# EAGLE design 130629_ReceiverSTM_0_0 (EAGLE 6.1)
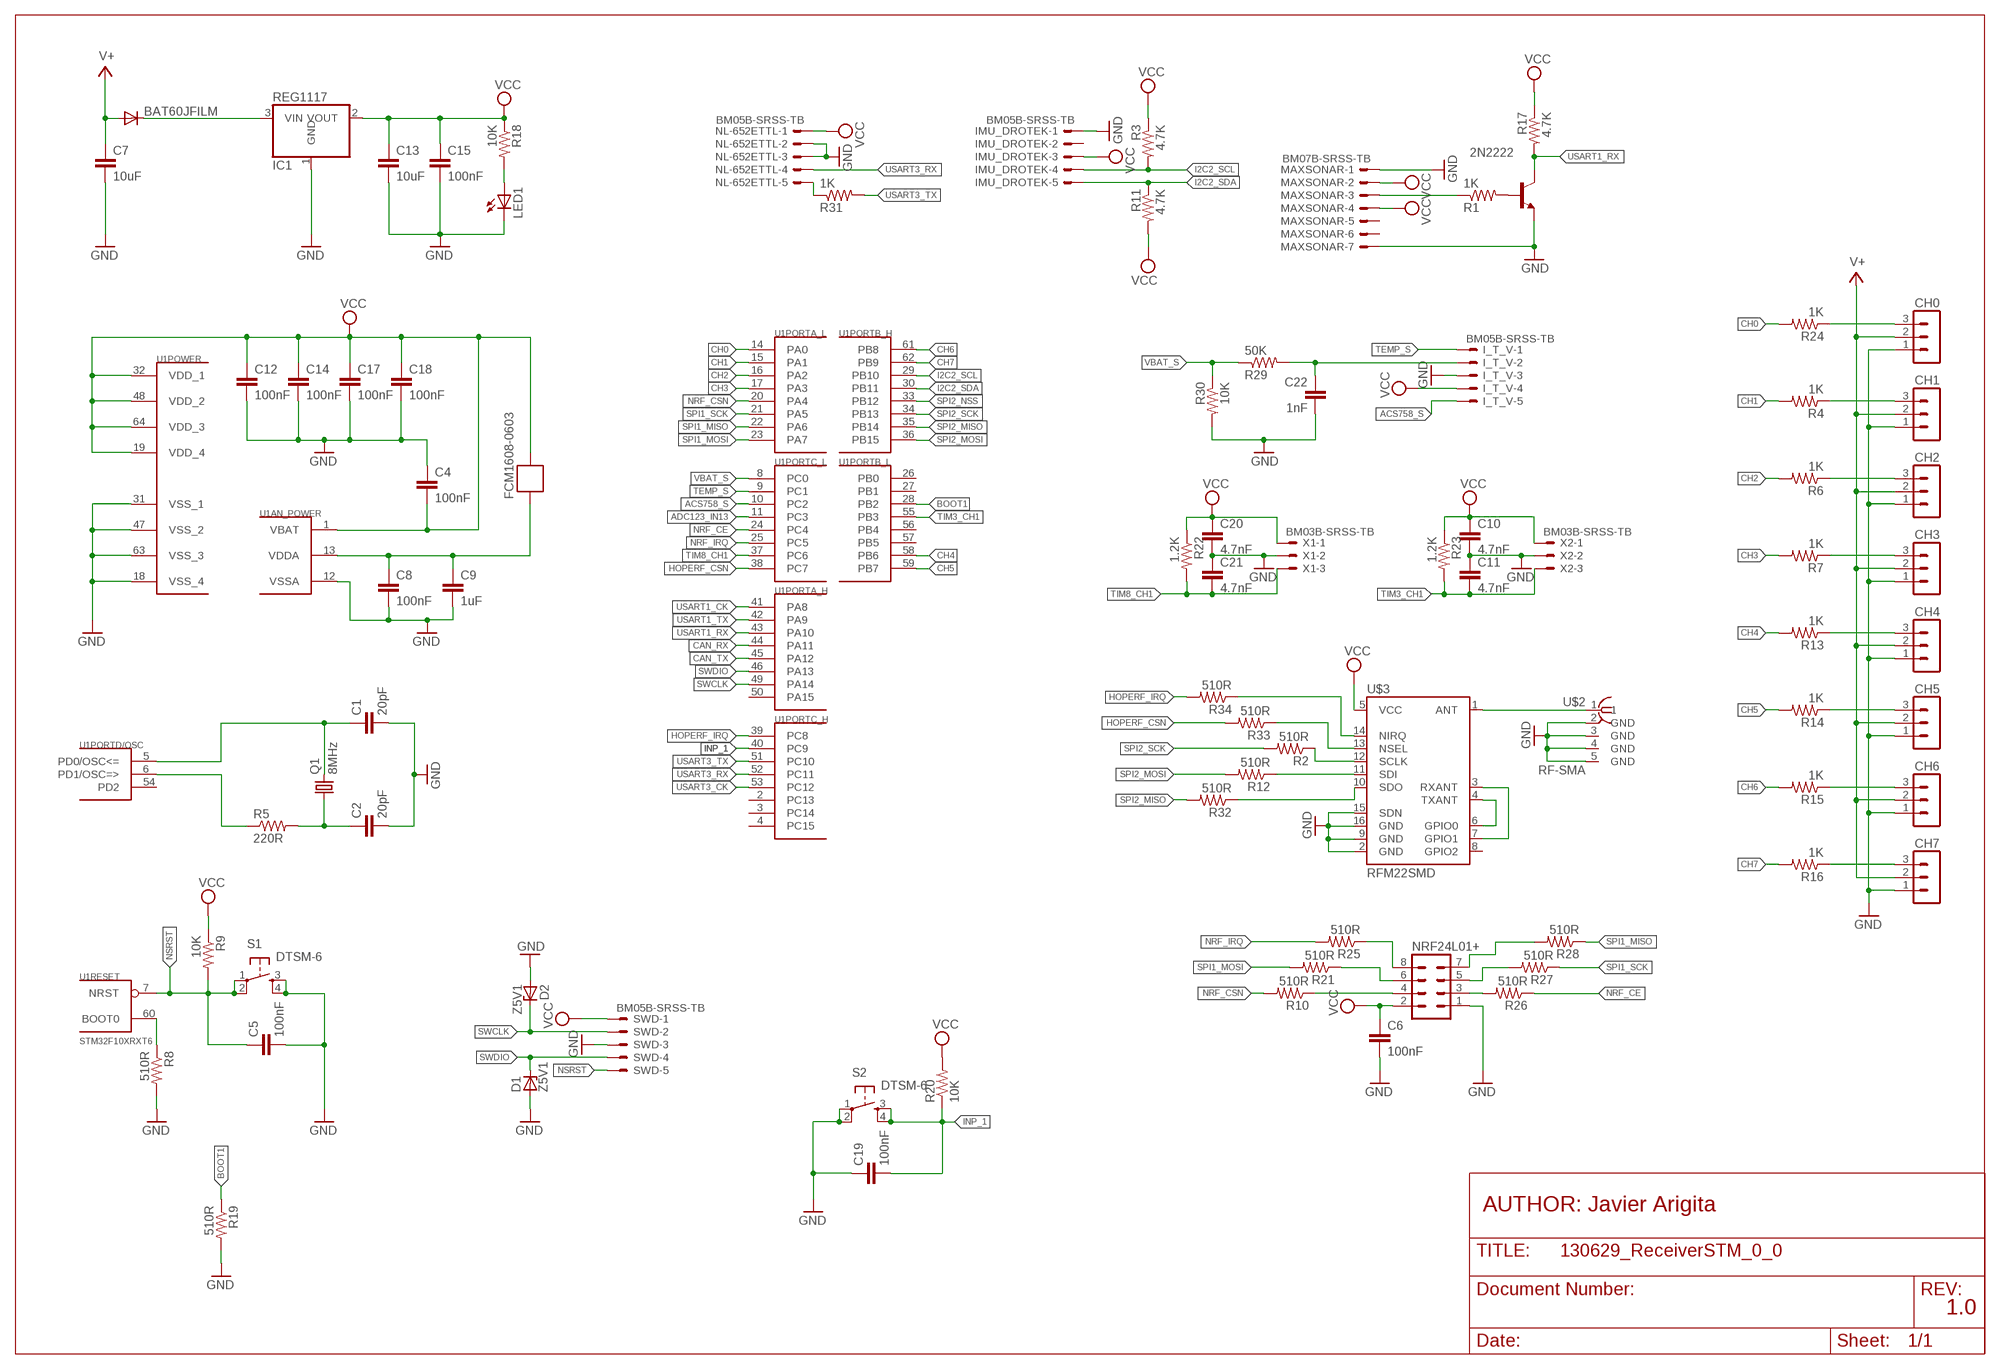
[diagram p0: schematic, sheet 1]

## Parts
2N2222  MMBT2222ALT1-NPN-SOT23-BEC  [SOT23-BEC]
BAT60JFILM  DIODE-SOD323-R  [SOD323-R]
C1  20pF  C-EUC0805  [C0805]
C2  20pF  C-EUC0805  [C0805]
C4  100nF  C-EUC0805  [C0805]
C5  100nF  C-EUC0805  [C0805]
C6  100nF  C-EUC0805  [C0805]
C7  10uF  C-EUC3216  [C3216]
C8  100nF  C-EUC0805  [C0805]
C9  1uF  C-EUC3216  [C3216]
C10  4.7nF  C-EUC0805  [C0805]
C11  4.7nF  C-EUC0805  [C0805]
C12  100nF  C-EUC0805  [C0805]
C13  10uF  C-EUC3216  [C3216]
C14  100nF  C-EUC0805  [C0805]
C15  100nF  C-EUC0805  [C0805]
C17  100nF  C-EUC0805  [C0805]
C18  100nF  C-EUC0805  [C0805]
C19  100nF  C-EUC0805  [C0805]
C20  4.7nF  C-EUC0805  [C0805]
C21  4.7nF  C-EUC0805  [C0805]
C22  1nF  C-EUC0805  [C0805]
CH0  MA03-1  [MA03-1]
CH1  MA03-1  [MA03-1]
CH2  MA03-1  [MA03-1]
CH3  MA03-1  [MA03-1]
CH4  MA03-1  [MA03-1]
CH5  MA03-1  [MA03-1]
CH6  MA03-1  [MA03-1]
CH7  MA03-1  [MA03-1]
D1  Z5V1  ZENER-DIODESOD80C  [SOD80C]
D2  Z5V1  ZENER-DIODESOD80C  [SOD80C]
FCM1608-0603  FERRITE-BEAD  [R0603]
I_T_V  BM05B-SRSS-TB  [BM05B-SRSS-TB]
IC1  REG1117  [SOT223]
IMU_DROTEK  BM05B-SRSS-TB  [BM05B-SRSS-TB]
LED1  LED0805  [CHIPLED_0805]
MAXSONAR  BM07B-SRSS-TB  [BM07B-SRSS-TB]
NL-652ETTL  BM05B-SRSS-TB  [BM05B-SRSS-TB]
NRF24L01+  MA04-2  [MA04-2]
Q1  8MHz  CRYSTALSM49  [SM49]
R1  1K  RESISTOR0805  [R0805]
R2  510R  RESISTOR0805  [R0805]
R3  4.7K  RESISTOR0805  [R0805]
R4  1K  RESISTOR0805  [R0805]
R5  220R  RESISTOR0805  [R0805]
R6  1K  RESISTOR0805  [R0805]
R7  1K  RESISTOR0805  [R0805]
R8  510R  RESISTOR0805  [R0805]
R9  10K  RESISTOR0805  [R0805]
R10  510R  RESISTOR0805  [R0805]
R11  4.7K  RESISTOR0805  [R0805]
R12  510R  RESISTOR0805  [R0805]
R13  1K  RESISTOR0805  [R0805]
R14  1K  RESISTOR0805  [R0805]
R15  1K  RESISTOR0805  [R0805]
R16  1K  RESISTOR0805  [R0805]
R17  4.7K  RESISTOR0805  [R0805]
R18  10K  RESISTOR0805  [R0805]
R19  510R  RESISTOR0805  [R0805]
R20  10K  RESISTOR0805  [R0805]
R21  510R  RESISTOR0805  [R0805]
R22  1.2K  RESISTOR0805  [R0805]
R23  1.2K  RESISTOR0805  [R0805]
R24  1K  RESISTOR0805  [R0805]
R25  510R  RESISTOR0805  [R0805]
R26  510R  RESISTOR0805  [R0805]
R27  510R  RESISTOR0805  [R0805]
R28  510R  RESISTOR0805  [R0805]
R29  50K  RESISTOR0805  [R0805]
R30  10K  RESISTOR0805  [R0805]
R31  1K  RESISTOR0805  [R0805]
R32  510R  RESISTOR0805  [R0805]
R33  510R  RESISTOR0805  [R0805]
R34  510R  RESISTOR0805  [R0805]
S1  DTSM-6  [DTSM-6]
S2  DTSM-6  [DTSM-6]
SWD  BM05B-SRSS-TB  [BM05B-SRSS-TB]
U1  STM32F10XRXT6  [TQFP64]
U$2  RF-SMA  [BU-SMA-H]
U$3  RFM22SMD  [RFM22-XXX-S2]
X1  BM03B-SRSS-TB  [BM03B-SRSS-TB]
X2  BM03B-SRSS-TB  [BM03B-SRSS-TB]

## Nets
ACS758_S: I_T_V.5 U1.10(PORTC_L:PC2)
ADC123_IN13: U1.11(PORTC_L:PC3)
BOOT1: R19.1 U1.28(PORTB_L:PB2)
CAN_RX: U1.44(PORTA_H:PA11)
CAN_TX: U1.45(PORTA_H:PA12)
CH0: R24.2 U1.14(PORTA_L:PA0)
CH1: R4.2 U1.15(PORTA_L:PA1)
CH2: R6.2 U1.16(PORTA_L:PA2)
CH3: R7.2 U1.17(PORTA_L:PA3)
CH4: R13.2 U1.58(PORTB_L:PB6)
CH5: R14.2 U1.59(PORTB_L:PB7)
CH6: R15.2 U1.61(PORTB_H:PB8)
CH7: R16.2 U1.62(PORTB_H:PB9)
GND: 2N2222.E C1.2 C2.2 C4.1 C5.2 C6.2 C7.2 C8.2 C9.2 C10.2 C11.1 C12.2 C13.2 C14.2 C15.2 C17.2 C18.2 C19.1 C20.2 C21.1 C22.2 CH0.1 CH1.1 CH2.1 CH3.1 CH4.1 CH5.1 CH6.1 CH7.1 D1.A D2.A I_T_V.3 IC1.1(GND) IMU_DROTEK.1 LED1.C MAXSONAR.1 MAXSONAR.7 NL-652ETTL.2 NL-652ETTL.3 NRF24L01+.1 R8.2 R19.2 R30.2 S1.3 S1.4 S2.1 S2.2 SWD.3 U1.12(AN_POWER:VSSA) U1.18(POWER:VSS_4) U1.31(POWER:VSS_1) U1.47(POWER:VSS_2) U1.63(POWER:VSS_3) U$2.2(GND) U$2.3(GND) U$2.4(GND) U$2.5(GND) U$3.2(GND) U$3.9(GND) U$3.15(SDN) U$3.16(GND) X1.2 X2.2
HOPERF_CSN: R33.1 R33.2 U1.38(PORTC_L:PC7) U$3.13(NSEL)
HOPERF_IRQ: R34.2 U1.39(PORTC_H:PC8)
I2C2_SCL: IMU_DROTEK.4 R3.2 U1.29(PORTB_H:PB10)
I2C2_SDA: IMU_DROTEK.5 R11.1 U1.30(PORTB_H:PB11)
INP_1: C19.2 R20.1 S2.3 S2.4 U1.40(PORTC_H:PC9)
N$1: C1.1 Q1.2 U1.5(PORTD/OSC:PD0/OSC<=)
N$2: R5.1 U1.6(PORTD/OSC:PD1/OSC=>)
N$3: C2.1 Q1.1 R5.2
N$4: R8.1 U1.60(RESET:BOOT0)
N$5: U$3.3(RXANT) U$3.7(GPIO1)
N$7: R2.1 U$3.12(SCLK)
N$8: R12.1 U$3.11(SDI)
N$9: CH0.3 R24.1
N$10: LED1.A R18.2
N$11: NL-652ETTL.5 R31.1
N$12: R32.1 U$3.10(SDO)
N$13: BAT60JFILM.C IC1.3(VIN)
N$14: MAXSONAR.3 R1.1
N$15: C22.1 I_T_V.2 R29.2
N$16: 2N2222.B R1.2
N$17: C8.1 C9.1 FCM1608-0603.2 U1.13(AN_POWER:VDDA)
N$18: NRF24L01+.4 R10.1
N$19: NRF24L01+.3 R26.2
N$20: U$2.1
N$21: CH2.3 R6.1
N$22: R34.1 U$3.14(NIRQ)
N$23: CH4.3 R13.1
N$31: CH3.3 R7.1
N$32: CH6.3 R15.1
N$34: CH5.3 R14.1
N$35: CH7.3 R16.1
N$36: NRF24L01+.5 R27.2
N$38: NRF24L01+.6 R21.1
N$39: NRF24L01+.8 R25.1
N$42: NRF24L01+.7 R28.2
N$53: CH1.3 R4.1
NRF_CE: R26.1 U1.24(PORTC_L:PC4)
NRF_CSN: R10.2 U1.20(PORTA_L:PA4)
NRF_IRQ: R25.2 U1.25(PORTC_L:PC5)
NSRST: C5.1 R9.2 S1.1 S1.2 SWD.5 U1.7(RESET:NRST)
SPI1_MISO: R28.1 U1.22(PORTA_L:PA6)
SPI1_MOSI: R21.2 U1.23(PORTA_L:PA7)
SPI1_SCK: R27.1 U1.21(PORTA_L:PA5)
SPI2_MISO: R32.2 U1.35(PORTB_H:PB14)
SPI2_MOSI: R12.2 U1.36(PORTB_H:PB15)
SPI2_NSS: U1.33(PORTB_H:PB12)
SPI2_SCK: R2.2 U1.34(PORTB_H:PB13)
SWCLK: D2.C SWD.2 U1.49(PORTA_H:PA14)
SWDIO: D1.C SWD.4 U1.46(PORTA_H:PA13)
TEMP_S: I_T_V.1 U1.9(PORTC_L:PC1)
TIM3_CH1: C11.2 R23.2 U1.55(PORTB_L:PB3) X2.3
TIM8_CH1: C21.2 R22.2 U1.37(PORTC_L:PC6) X1.3
USART1_CK: U1.41(PORTA_H:PA8)
USART1_RX: 2N2222.C R17.2 U1.43(PORTA_H:PA10)
USART1_TX: U1.42(PORTA_H:PA9)
USART3_CK: U1.53(PORTC_H:PC12)
USART3_RX: NL-652ETTL.4 U1.52(PORTC_H:PC11)
USART3_TX: R31.2 U1.51(PORTC_H:PC10)
V+: BAT60JFILM.A C7.1 CH0.2 CH1.2 CH2.2 CH3.2 CH4.2 CH5.2 CH6.2 CH7.2
VBAT_S: R29.1 R30.1 U1.8(PORTC_L:PC0)
VCC: C4.2 C6.1 C10.1 C12.1 C13.1 C14.1 C15.1 C17.1 C18.1 C20.1 FCM1608-0603.1 I_T_V.4 IC1.2(VOUT) IMU_DROTEK.3 MAXSONAR.2 MAXSONAR.4 NL-652ETTL.1 NRF24L01+.2 R3.1 R9.1 R11.2 R17.1 R18.1 R20.2 R22.1 R23.1 SWD.1 U1.1(AN_POWER:VBAT) U1.19(POWER:VDD_4) U1.32(POWER:VDD_1) U1.48(POWER:VDD_2) U1.64(POWER:VDD_3) U$3.5(VCC) X1.1 X2.1
Unconnected: IMU_DROTEK.2 MAXSONAR.5 MAXSONAR.6 U1.2(PORTC_H:PC13) U1.3(PORTC_H:PC14) U1.4(PORTC_H:PC15) U1.26(PORTB_L:PB0) U1.27(PORTB_L:PB1) U1.50(PORTA_H:PA15) U1.54(PORTD/OSC:PD2) U1.56(PORTB_L:PB4) U1.57(PORTB_L:PB5) U$3.1(ANT) U$3.4(TXANT) U$3.6(GPIO0) U$3.8(GPIO2)

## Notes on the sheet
- AUTHOR: Javier Arigita
- 1.0

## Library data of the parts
2N2222 = transistor:*-NPN-: NPN Transistror BF959 corrected 2008.03.06
BAT60JFILM = diode:DIODE-: DIODE
C1 C2 C4-C6 C8 C10-C12 C14 C15 C17-C22 = rcl:C-EU: CAPACITOR, European symbol
C7 C9 C13 = resistor:C-EU: CAPACITOR, European symbol
CH0 CH1-CH7 = con-lstb:MA03-1: PIN HEADER; OC_FARNELL: unknown; OC_NEWARK: unknown
D1 D2 = diode:ZENER-DIODE: Z-Diode
FCM1608-0603 = BaseApp:FERRITE-BEAD
I_T_V IMU_DROTEK NL-652ETTL SWD = con-jst2:?M05B-SRSS-TB: Disconnectable Crimp style connector, 1.0mm pitch 5 contacts
IC1 = CEDT:REG1117: 800mA and 1A Low Dropout (LDO) Positive Regulator 1.8V, 2.5V, 2.85V, 3.3V, 5V, and Adj
LED1 = CEDT:LED
MAXSONAR = con-jst2:?M07B-SRSS-TB: Disconnectable Crimp style connector, 1.0mm pitch 7 contacts
NRF24L01+ = con-lstb:MA04-2: PIN HEADER; OC_FARNELL: unknown; OC_NEWARK: unknown
Q1 = crystal:CRYSTAL: CRYSTAL; OC_FARNELL: unknown; OC_NEWARK: unknown
R1-R34 = CEDT:RESISTOR
S1 S2 = switch-tact:DTSM-6
U1 = stm32:STM32F10XRXT6: STM32F101/103 64pin LQFP
U$2 = BaseApp:RF-SMA
U$3 = SparkFun-RF:RFM22: The RFM22 is a low-power, low cost radio that is capable of operating in the 434MHz and 900MHz open bands. It's frequency is software defined and there are some very good libraries written for it.
X1 X2 = con-jst2:?M03B-SRSS-TB: Disconnectable Crimp style connector, 1.0mm pitch 3 contacts

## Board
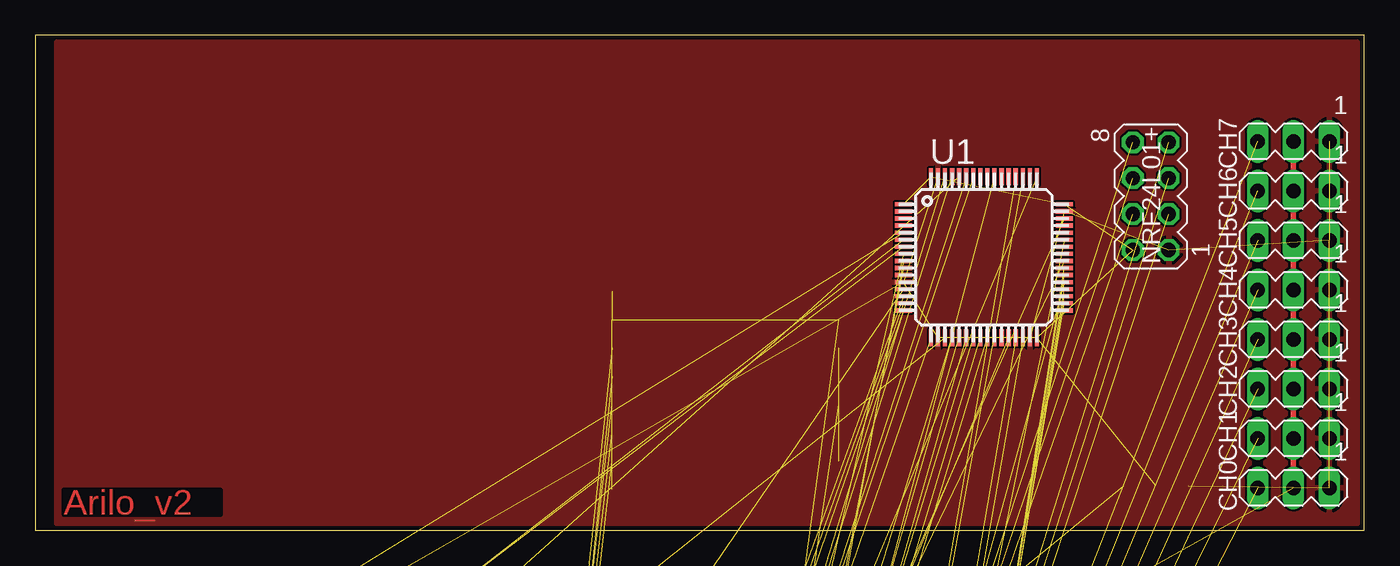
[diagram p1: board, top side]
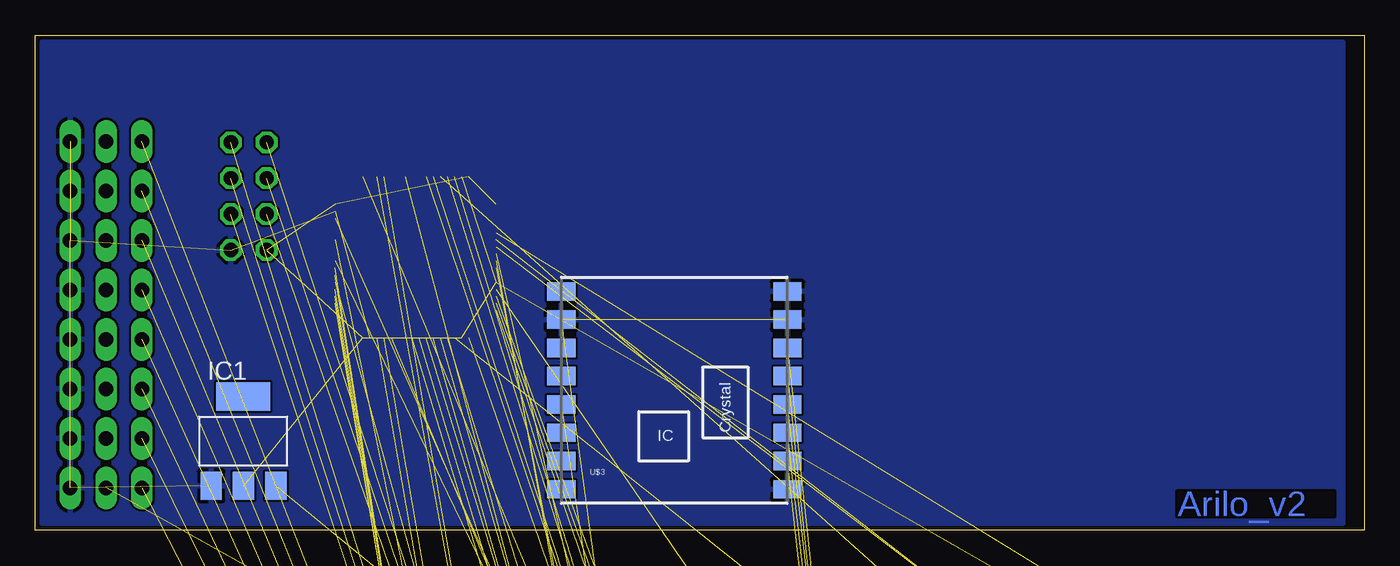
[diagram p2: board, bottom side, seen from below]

Size 94 x 35 mm. Coordinates in mm from the lower left corner, seen from the top.
Outline: 0,0 94,0 94,35 0,35 0,0
Copper layers (1*16): Top 0.035mm / dielectric 1.5mm / Bottom 0.035mm
Design rules: minimum track width 6mil, minimum drill 12mil, track to track 6mil, track to pad 6mil, pad to pad 6mil, via to via 6mil, smd to smd 0mil, copper to edge 10mil, drill to drill 10mil, minimum pad ring 10mil, minimum via ring 6mil, stop-mask expansion 2mil, vias tented up to drill 100mil, thermal gap 10mil

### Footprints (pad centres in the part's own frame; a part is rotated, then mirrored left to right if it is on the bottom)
SOT23-BEC = smd 1 x 1.4: B -0.95,-1.1; C 0,1.1; E 0.95,-1.1
SOD323-R = smd 0.6 x 0.6: A 1.1,0; C -1.1,0
C0805 = smd 1.3 x 1.5: 1 -0.95,0; 2 0.95,0
C3216 = smd 1.6 x 1.8: 1 -1.4,0; 2 1.4,0
MA03-1 = drill 1.016 long: 1 -2.54,0; 2 0,0; 3 2.54,0
SOD80C = smd 1.4 x 1.8: A 1.7,0; C -1.7,0
R0603 = smd 1 x 1.1: 1 -0.85,0; 2 0.85,0
BM05B-SRSS-TB = smd 0.6 x 1.55: 1 2,-1.625; 2 1,-1.625; 3 0,-1.625; 4 -1,-1.625; 5 -2,-1.625 | smd 1.2 x 1.8: FIT@1 3.3,0.9; FIT@2 -3.3,0.9
SOT223 = smd 1.499 x 2.007: 1 -2.261,-3.15; 2 0.025,-3.15; 3 2.311,-3.15 | smd 3.81 x 2.007: 4 0,3.15
CHIPLED_0805 = smd 1.2 x 1.2: A 0,-1.05; C 0,1.05
BM07B-SRSS-TB = smd 0.6 x 1.55: 1 3,-1.625; 2 2,-1.625; 3 1,-1.625; 4 0,-1.625; 5 -1,-1.625; 6 -2,-1.625; 7 -3,-1.625 | smd 1.2 x 1.8: FIT@1 4.3,0.9; FIT@2 -4.3,0.9
MA04-2 = drill 1.016 octagon: 1 -3.81,-1.27; 2 -3.81,1.27; 3 -1.27,-1.27; 4 -1.27,1.27; 5 1.27,-1.27; 6 1.27,1.27; 7 3.81,-1.27; 8 3.81,1.27
SM49 = smd 5.08 x 1.778: 1 -4.826,0; 2 4.826,0
R0805 = smd 1.3 x 1.5: 1 -0.95,0; 2 0.95,0
DTSM-6 = smd 1.55 x 1.3: 1 -3.975,2.25; 2 3.975,2.25; 3 -3.975,-2.25; 4 3.975,-2.25
TQFP64 = smd 1.2 x 0.3: 1 -5.7,3.75; 2 -5.7,3.25; 3 -5.7,2.75; 4 -5.7,2.25; 5 -5.7,1.75; 6 -5.7,1.25; 7 -5.7,0.75; 8 -5.7,0.25; 9 -5.7,-0.25; 10 -5.7,-0.75; 11 -5.7,-1.25; 12 -5.7,-1.75; 13 -5.7,-2.25; 14 -5.7,-2.75; 15 -5.7,-3.25; 16 -5.7,-3.75; 33 5.7,-3.75; 34 5.7,-3.25; 35 5.7,-2.75; 36 5.7,-2.25; 37 5.7,-1.75; 38 5.7,-1.25; 39 5.7,-0.75; 40 5.7,-0.25; 41 5.7,0.25; 42 5.7,0.75; 43 5.7,1.25; 44 5.7,1.75; 45 5.7,2.25; 46 5.7,2.75; 47 5.7,3.25; 48 5.7,3.75 | smd 0.3 x 1.2: 17 -3.75,-5.7; 18 -3.25,-5.7; 19 -2.75,-5.7; 20 -2.25,-5.7; 21 -1.75,-5.7; 22 -1.25,-5.7; 23 -0.75,-5.7; 24 -0.25,-5.7; 25 0.25,-5.7; 26 0.75,-5.7; 27 1.25,-5.7; 28 1.75,-5.7; 29 2.25,-5.7; 30 2.75,-5.7; 31 3.25,-5.7; 32 3.75,-5.7; 49 3.75,5.7; 50 3.25,5.7; 51 2.75,5.7; 52 2.25,5.7; 53 1.75,5.7; 54 1.25,5.7; 55 0.75,5.7; 56 0.25,5.7; 57 -0.25,5.7; 58 -0.75,5.7; 59 -1.25,5.7; 60 -1.75,5.7; 61 -2.25,5.7; 62 -2.75,5.7; 63 -3.25,5.7; 64 -3.75,5.7
BU-SMA-H = drill 1.5: 1 0,0 | drill 1.6: 2 -2.54,2.54; 3 2.54,2.54; 4 2.54,-2.54; 5 -2.54,-2.54
RFM22-XXX-S2 = smd 2 x 1.3: 1 -8,7; 2 -8,5; 3 -8,3; 4 -8,1; 5 -8,-1; 6 -8,-3; 7 -8,-5; 8 -8,-7; 9 8,-7; 10 8,-5; 11 8,-3; 12 8,-1; 13 8,1; 14 8,3; 15 8,5; 16 8,7
BM03B-SRSS-TB = smd 0.6 x 1.55: 1 1,-1.625; 2 0,-1.625; 3 -1,-1.625 | smd 1.2 x 1.8: FIT@1 2.3,0.9; FIT@2 -2.3,0.9

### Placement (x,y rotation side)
2N2222  not placed on the board
BAT60JFILM  not placed on the board
C1  not placed on the board
C2  not placed on the board
C4  not placed on the board
C5  not placed on the board
C6  not placed on the board
C7  not placed on the board
C8  not placed on the board
C9  not placed on the board
C10  not placed on the board
C11  not placed on the board
C12  not placed on the board
C13  not placed on the board
C14  not placed on the board
C15  not placed on the board
C17  not placed on the board
C18  not placed on the board
C19  not placed on the board
C20  not placed on the board
C21  not placed on the board
C22  not placed on the board
CH0  89,3 180 top
CH1  89,6.5 180 top
CH2  89,10 180 top
CH3  89,13.5 180 top
CH4  89,17 180 top
CH5  89,20.5 180 top
CH6  89,24 180 top
CH7  89,27.5 180 top
D1  not placed on the board
D2  not placed on the board
FCM1608-0603  not placed on the board
I_T_V  not placed on the board
IC1  79.3,6.3 0 bottom
IMU_DROTEK  not placed on the board
LED1  not placed on the board
MAXSONAR  not placed on the board
NL-652ETTL  not placed on the board
NRF24L01+  78.91,23.63 90 top
Q1  not placed on the board
R1  not placed on the board
R2  not placed on the board
R3  not placed on the board
R4  not placed on the board
R5  not placed on the board
R6  not placed on the board
R7  not placed on the board
R8  not placed on the board
R9  not placed on the board
R10  not placed on the board
R11  not placed on the board
R12  not placed on the board
R13  not placed on the board
R14  not placed on the board
R15  not placed on the board
R16  not placed on the board
R17  not placed on the board
R18  not placed on the board
R19  not placed on the board
R20  not placed on the board
R21  not placed on the board
R22  not placed on the board
R23  not placed on the board
R24  not placed on the board
R25  not placed on the board
R26  not placed on the board
R27  not placed on the board
R28  not placed on the board
R29  not placed on the board
R30  not placed on the board
R31  not placed on the board
R32  not placed on the board
R33  not placed on the board
R34  not placed on the board
S1  not placed on the board
S2  not placed on the board
SWD  not placed on the board
U1  67.1,19.3 0 top
U$2  not placed on the board
U$3  48.8,9.9 0 bottom
X1  not placed on the board
X2  not placed on the board

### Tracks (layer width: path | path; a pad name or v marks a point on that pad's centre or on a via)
ACS758_S  (1 unrouted)
BOOT1  (1 unrouted)
CH0  (1 unrouted)
CH1  (1 unrouted)
CH2  (1 unrouted)
CH3  (1 unrouted)
CH4  (1 unrouted)
CH5  (1 unrouted)
CH6  (1 unrouted)
CH7  (1 unrouted)
GND  (62 unrouted)
  pour Top: 1.5,34.5 93.5,34.5 93.5,0.5 1.5,0.5
  pour Bottom: 1.5,34.5 93.5,34.5 93.5,0.5 1.5,0.5
HOPERF_CSN  (3 unrouted)
HOPERF_IRQ  (1 unrouted)
I2C2_SCL  (2 unrouted)
I2C2_SDA  (2 unrouted)
INP_1  (4 unrouted)
N$1  (2 unrouted)
N$2  (1 unrouted)
N$3  (2 unrouted)
N$4  (1 unrouted)
N$5  (1 unrouted)
N$7  (1 unrouted)
N$8  (1 unrouted)
N$9  (1 unrouted)
N$10  (1 unrouted)
N$11  (1 unrouted)
N$12  (1 unrouted)
N$13  (1 unrouted)
N$14  (1 unrouted)
N$15  (2 unrouted)
N$16  (1 unrouted)
N$17  (3 unrouted)
N$18  (1 unrouted)
N$19  (1 unrouted)
N$21  (1 unrouted)
N$22  (1 unrouted)
N$23  (1 unrouted)
N$31  (1 unrouted)
N$32  (1 unrouted)
N$34  (1 unrouted)
N$35  (1 unrouted)
N$36  (1 unrouted)
N$38  (1 unrouted)
N$39  (1 unrouted)
N$42  (1 unrouted)
N$53  (1 unrouted)
NRF_CE  (1 unrouted)
NRF_CSN  (1 unrouted)
NRF_IRQ  (1 unrouted)
NSRST  (5 unrouted)
SPI1_MISO  (1 unrouted)
SPI1_MOSI  (1 unrouted)
SPI1_SCK  (1 unrouted)
SPI2_MISO  (1 unrouted)
SPI2_MOSI  (1 unrouted)
SPI2_SCK  (1 unrouted)
SWCLK  (2 unrouted)
SWDIO  (2 unrouted)
TEMP_S  (1 unrouted)
TIM3_CH1  (3 unrouted)
TIM8_CH1  (3 unrouted)
USART1_RX  (2 unrouted)
USART3_RX  (1 unrouted)
USART3_TX  (1 unrouted)
V+  (2 unrouted)
  Top 0.406: CH7.2 CH6.2 CH5.2 CH4.2 CH3.2 CH2.2 CH1.2 CH0.2
VBAT_S  (2 unrouted)
VCC  (34 unrouted)

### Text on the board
Top: Arilo_v2
Bottom: Arilo_v2

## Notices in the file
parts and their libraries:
SparkFun-RF: Licensing: CC v3.0 Share-Alike You are welcome to use this library for commercial purposes.
